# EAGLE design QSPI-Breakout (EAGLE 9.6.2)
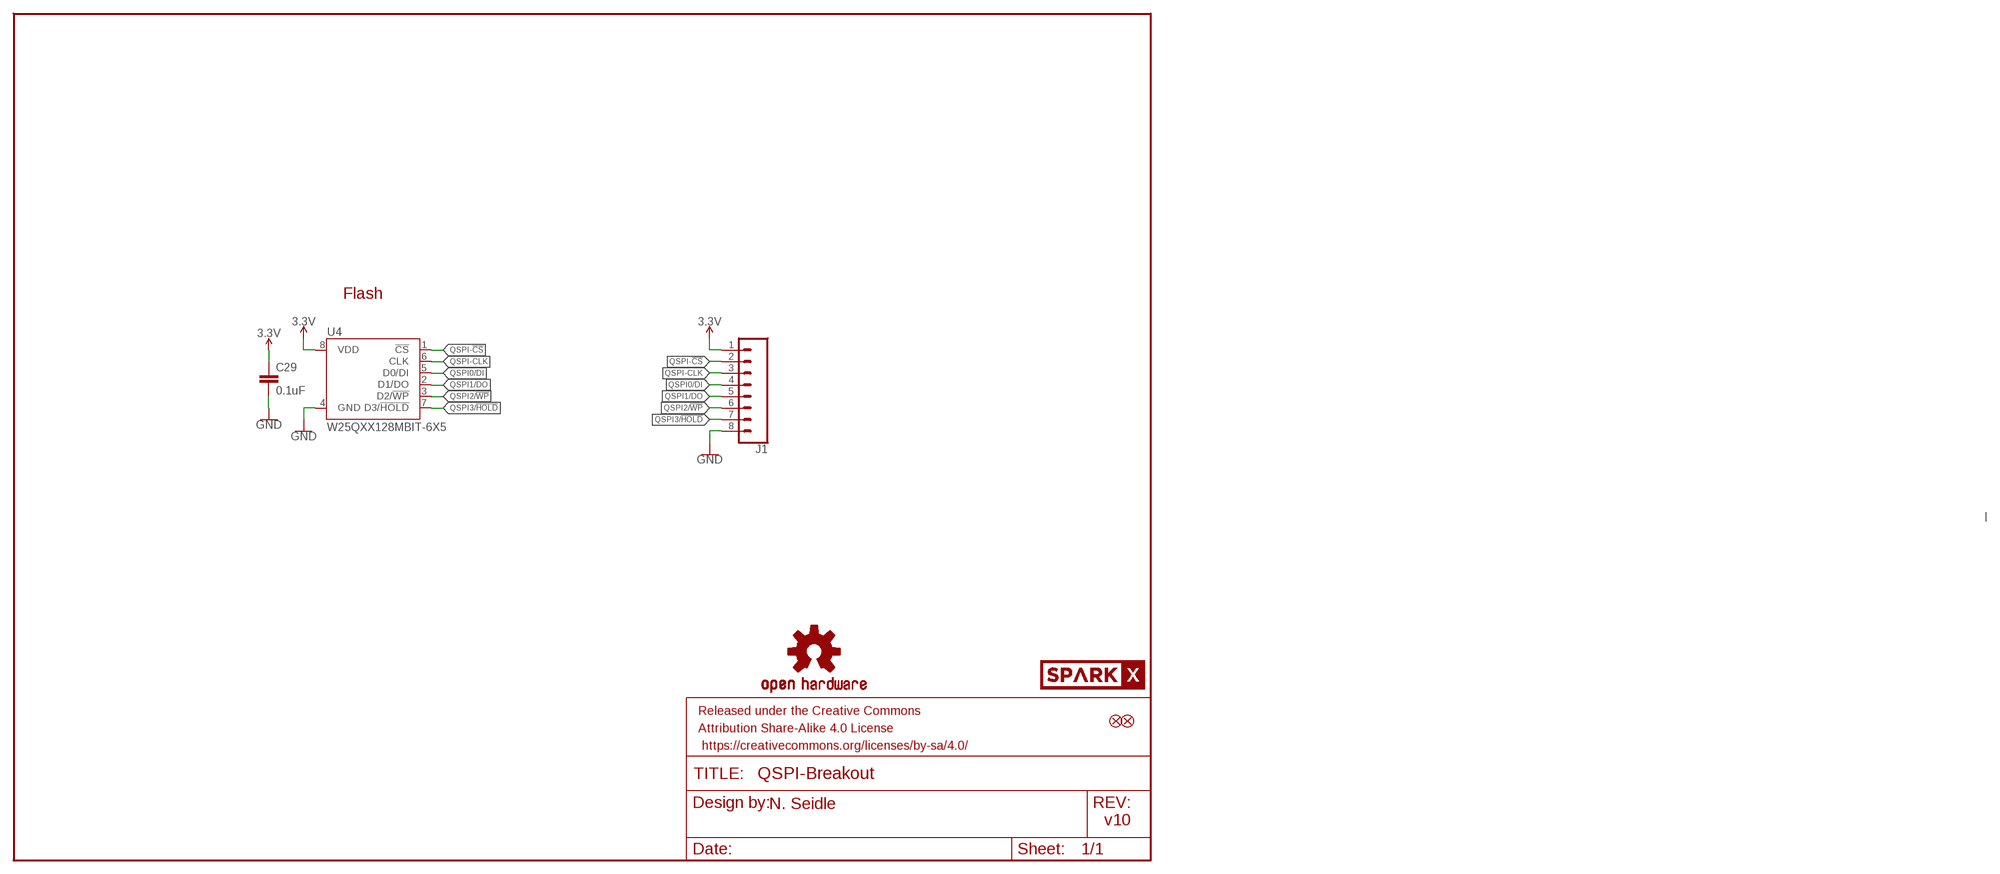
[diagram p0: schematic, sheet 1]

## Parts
C29  0.1uF  0.1UF-0603-25V-(+80/-20%)  [0603]
FD1  FIDUCIALUFIDUCIAL  [FIDUCIAL-MICRO]
FD2  FIDUCIALUFIDUCIAL  [FIDUCIAL-MICRO]
FRAME2  FRAME-LETTER  [CREATIVE_COMMONS]
J1  CONN_08NO_SILK_DNP  [1X08_NO_SILK]
LOGO2  OSHW-LOGONO_SILK  [DUMMY]
U4  W25QXX128MBIT-6X5  W25QXX128MBIT-6X5-SKINNY_CENTER  [WSON-8-6X5-SKINNY_CENTERPAD]
U$3  SPARKX-LOGO4  [SPARKX-MEDIUM]

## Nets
3.3V: C29.1 J1.1 U4.8(VDD)
GND: C29.2 J1.8 U4.4(GND)
QSPI0/DI: J1.4 U4.5(D0/DI)
QSPI1/DO: J1.5 U4.2(D1/DO)
QSPI2/!WP!: J1.6 U4.3(D2/!WP!)
QSPI3/!HOLD!: J1.7 U4.7(D3/!HOLD!)
QSPI-!CS!: J1.2 U4.1(!CS!)
QSPI-CLK [Clock]: J1.3 U4.6(CLK)

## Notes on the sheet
- Flash
- N. Seidle
- v10

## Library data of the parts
C29 = SparkFun-Capacitors:0.1UF: 0.1µF ceramic capacitors; PROD_ID: CAP-00810
FD1 FD2 = SparkFun-Aesthetics:FIDUCIAL: Fiducial Alignment Points
FRAME2 = SparkFun-Aesthetics:FRAME-LETTER: Schematic Frame - Letter
J1 = SparkFun-Connectors:CONN_08: Multi connection point. Often used as Generic Header-pin footprint for 0.1 inch spaced/style header connections On any of the 0.1 inch spaced packages, you can populate with these: Break Away Headers - Straight (PRT-00116) Break Away Male Headers - Right Angle (PRT-00553) Female Headers (PRT-00115)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
LOGO2 = SparkFun-Aesthetics:OSHW-LOGO: Open-Source Hardware (OSHW) Logo
U4 = SparkFun-MicroMod:W25QXX; PROD_ID: IC-15107
U$3 = SparkX:SPARKX-LOGO

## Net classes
1 90Ohm: width 0.114 mm, clearance 0.127 mm
2 Clock: width 0.089 mm, clearance 0.178 mm
3 DCBoost: width 0.381 mm

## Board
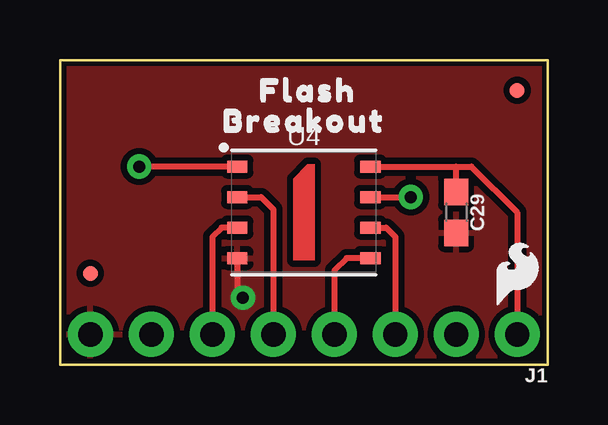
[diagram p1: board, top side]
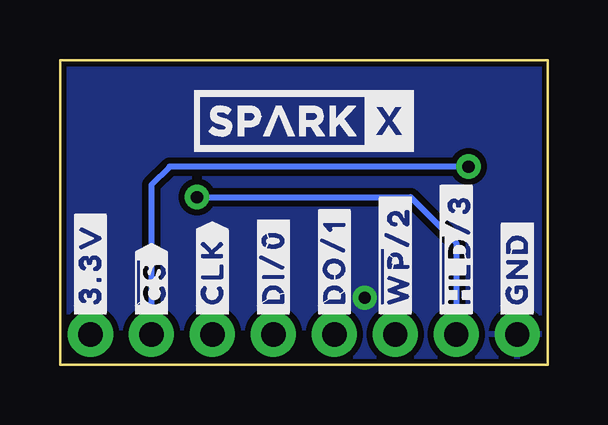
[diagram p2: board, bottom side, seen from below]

Size 20.32 x 12.7 mm. Coordinates in mm from the lower left corner, seen from the top.
Outline: 20.32,0 0,0 0,12.7 20.32,12.7 20.32,0
Copper layers (1*16): Top 0.035mm / dielectric 1.5mm / Bottom 0.035mm
Design rules "SparkFun-2-layer-STANDARD": minimum track width 10mil, minimum drill 20mil, track to track 10mil, track to pad 8mil, pad to pad 8mil, via to via 10mil, smd to smd 8mil, copper to edge 8mil, drill to drill 8mil, minimum pad ring 10mil, minimum via ring 10mil, stop-mask expansion 4mil, vias tented up to drill 25mil, thermal gap 10mil

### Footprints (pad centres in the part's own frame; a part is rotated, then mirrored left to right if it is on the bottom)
0603 = smd 1.1 x 1: 1 -0.85,0; 2 0.85,0
FIDUCIAL-MICRO = smd 0.635 x 0.635: 1 0,0
1X08_NO_SILK = drill 1.016 pad 1.88: 1 0,0; 2 2.54,0; 3 5.08,0; 4 7.62,0; 5 10.16,0; 6 12.7,0; 7 15.24,0; 8 17.78,0
WSON-8-6X5-SKINNY_CENTERPAD = smd 0.85 x 0.5: 1 -2.775,1.905; 2 -2.775,0.635; 3 -2.775,-0.635; 4 -2.775,-1.905; 5 2.775,-1.905; 6 2.775,-0.635; 7 2.775,0.635; 8 2.775,1.905

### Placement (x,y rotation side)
C29  16.51,6.35 270 top
FD1  19.05,11.43 0 top
FD2  1.27,3.81 0 top
FRAME2  not placed on the board
J1  19.05,1.27 180 top
LOGO2  not placed on the board
U4  10.16,6.35 0 top
U$1  [BREAKOUT1]  6.1,10.16 0 top
U$2  [FLASH0]  7.62,11.43 0 top
U$3  10.16,10.16 0 bottom
U$4  [##HLD##3#2]  3.81,1.78 90 bottom
U$5  [##WP##2#3]  6.35,1.78 90 bottom
U$6  [SFE_LOGO_FLAME_.1]  19.05,3.81 0 top
U$7  [#3#3V#1]  19.05,1.78 90 bottom
U$8  [#CLK#6]  13.97,1.78 90 bottom
U$9  [#DI#0#5]  11.43,1.78 90 bottom
U$10  [#DO#1#4]  8.89,1.78 90 bottom
U$11  [#GND#0]  1.27,1.78 90 bottom
U$12  [##CS##7]  16.51,1.78 90 bottom

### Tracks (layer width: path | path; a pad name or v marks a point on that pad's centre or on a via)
3.3V
  Top 0.254: U4.8 16.51,8.26 | 16.51,8.26 17.14,8.26 19.05,6.35 J1.1 | C29.1 16.51,8.26
GND  (via drill 0.51)
  Top 0.254: U4.4 7.38,3.03 v7.62,2.79
  pour Bottom (isolate 0.203): 0,0 0,12.7 20.32,12.7 20.32,0
  pour Top (isolate 0.203): 0,0 0,12.7 20.32,12.7 20.32,0
QSPI0/DI
  Top 0.254: U4.5 11.94,4.45 11.43,3.94 J1.4
QSPI1/DO
  Top 0.254: U4.2 8.38,6.99 8.89,6.48 J1.5
QSPI2/!WP!
  Top 0.254: U4.3 6.73,5.71 6.35,5.33 J1.6
QSPI3/!HOLD!  (via drill 0.51)
  Top 0.254: U4.7 v14.61,6.99
  Bottom 0.254: v14.61,6.99 5.71,6.99 3.81,5.08 J1.7
QSPI-!CS!  (via drill 0.51)
  Top 0.254: U4.1 v3.3,8.26
  Bottom 0.254: v3.3,8.26 15.75,8.26 16.51,7.49 J1.2
QSPI-CLK
  Top 0.254: U4.6 13.59,5.71 13.97,5.33 J1.3

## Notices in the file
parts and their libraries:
SparkFun-Aesthetics: Licensing: Creative Commons ShareAlike 4.0 International - https://creativecommons.org/licenses/by-sa/4.0
SparkFun-Aesthetics: Released under the Creative Commons Attribution Share-Alike 4.0 License
SparkFun-Aesthetics: https://creativecommons.org/licenses/by-sa/4.0
